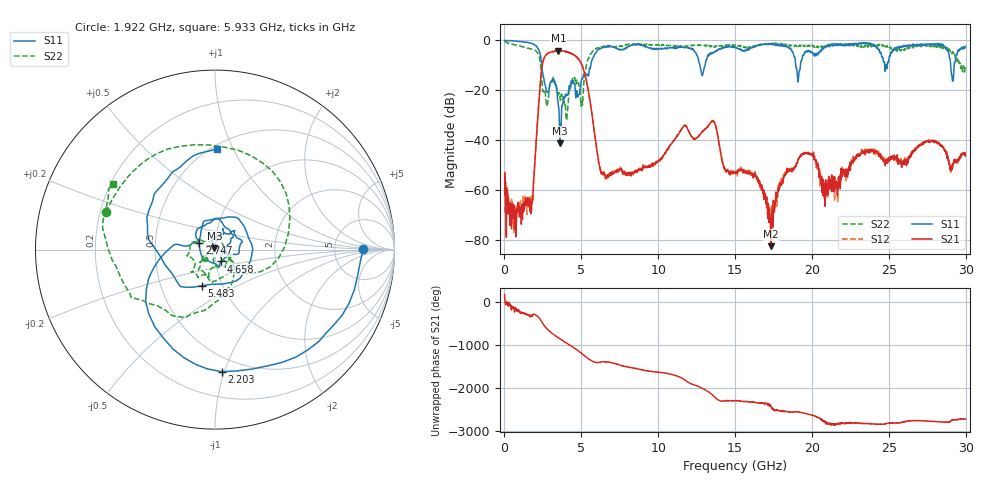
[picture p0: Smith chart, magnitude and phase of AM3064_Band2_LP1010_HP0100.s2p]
# Hz S DB R 50.0
!freq dBS11 angS11 dBS21 angS21 dBS12 angS12 dBS22 angS22
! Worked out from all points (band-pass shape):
!   1600 points, 10 MHz to 29.98 GHz, reference 50 ohm
!   highest |S21| = -4.05 dB at 3.515 GHz (marker M1); lowest = -82.3 dB at 17.35 GHz (marker M2)
!   |S21| within 3 dB of the highest: 2.578 GHz to 4.758 GHz (2.181 GHz wide, 59.5 % of centre)
!   lowest |S11| = -41.1 dB at 3.609 GHz (marker M3), VSWR 1.02, Z = 49.6 + j0.797 ohm
!   |S11| at or under -10 dB: 2.427 GHz to 5.619 GHz (3.192 GHz wide, 79.4 % of centre); 12.72 GHz to 13.05 GHz (329.9 MHz wide, 2.56 % of centre); 18.95 GHz to 19.25 GHz (303.9 MHz wide, 1.59 % of centre)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
!   |S22| runs from -31.5 to -0.2 dB; largest |S21 - S12| = 0.018
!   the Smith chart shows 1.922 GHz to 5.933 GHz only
!   S11 on the Smith chart (normalised r, x): 1.922 GHz: 10, +0; 2.203 GHz: 0.39, -0.98; 2.747 GHz: 0.84, +0.06; 4.658 GHz: 1.06, -0.14; 5.483 GHz: 0.80, -0.34; 5.933 GHz: 0.53, +0.86
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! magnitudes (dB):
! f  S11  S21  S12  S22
! 10 MHz  0.0  -53.1  -61.0  -0.2
! 722.3 MHz  -0.2  -67.8  -71.6  -1.8
! 1.922 GHz  -1.7  -54.5  -54.0  -3.8
! 2.203 GHz  -3.3  -27.8  -27.7  -5.3
! 2.747 GHz  -20.5  -5.5  -5.5  -26.0
! 3.515 GHz  -26.5  -4.1  -4.1  -21.8
! 3.609 GHz  -41.1  -4.3  -4.2  -22.5
! 4.658 GHz  -22.6  -6.5  -6.3  -17.2
! 5.015 GHz  -15.5  -9.5  -9.6  -24.5
! 5.483 GHz  -13.4  -21.2  -20.9  -7.2
! 5.933 GHz  -5.0  -40.4  -40.5  -3.4
! 6.664 GHz  -2.2  -53.9  -54.4  -2.3
! 10 GHz  -3.4  -48.2  -48.2  -1.8
! 13.54 GHz  -5.2  -32.3  -32.1  -2.6
! 15 GHz  -2.6  -52.9  -53.3  -1.8
! 17.35 GHz  -1.3  -82.3  -71.7  -1.2
! 19.99 GHz  -4.6  -45.4  -45.8  -1.9
! 20.82 GHz  -2.7  -61.1  -58.0  -2.3
! 25 GHz  -8.2  -47.2  -47.2  -2.3
! 28.39 GHz  -1.3  -41.9  -42.1  -3.1
! 29.18 GHz  -16.1  -49.6  -50.7  -4.7
! 29.98 GHz  -2.4  -46.2  -46.1  -10.2
